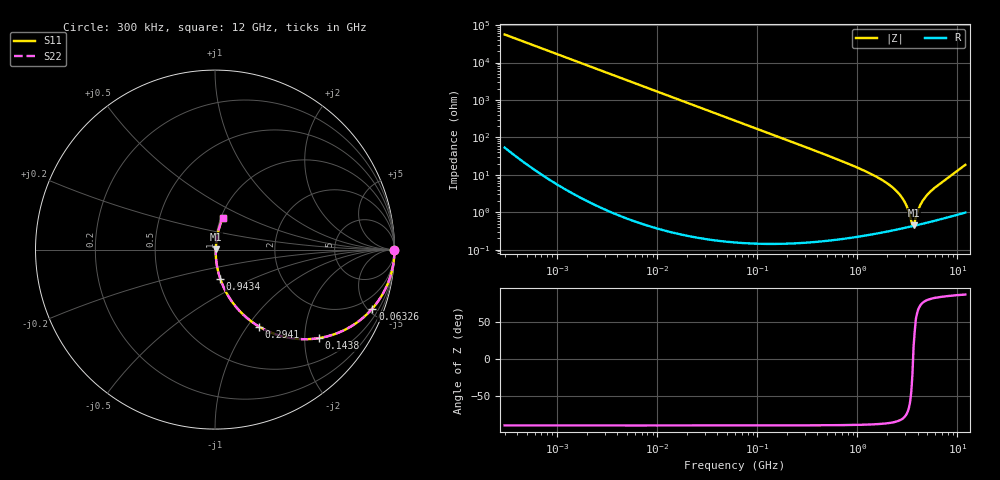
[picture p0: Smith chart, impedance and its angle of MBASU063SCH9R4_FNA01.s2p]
! MBASU063SCH9R4_FNA01  S-PARAMETER MODEL  ( General Type )
! Model Generated by TAIYO YUDEN Corporation (http://www.ty-top.com)
! Version 1.0
! TAIYO YUDEN Control No. 130801
! Copyright(c) 2013 TAIYO YUDEN CO.,LTD. All Rights Reserved.
! Product Description (link to TY-COMPAS)
! https://ds.yuden.co.jp/TYCOMPAS/or/detail?pn=MBASU063SCH9R4DFNA01&u=M
! Products Name : Multilayer Ceramic Capacitors
! Characteristics :
!  Capacitance : 9.4 pF , Rated Voltage : 50V , TCC : CH / C0H
!  Case Size : 0.6 x 0.3 / 0.024 x 0.012 [mm/inch] , Thickness : 0.3 / 0.012 [mm/inch]
!  (Conditions: Temperature = 25 degC , DC Bias Current/Voltage = 0A / 0V)
! External Node Assignments :
!  1  o---| |---o  2
! GND o---------o GND
! Frequency Range : 0.3MHz  -  12000MHz  [ 401 STEP ]
# MHz S RI R 50
! Freq[MHz].  S11 Real  S11 Imag  S21 Real  S21 Imag  S12 Real  S12 Imag  S22 Real  S22 Imag
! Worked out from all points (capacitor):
!   401 points, 300 kHz to 12 GHz, reference 50 ohm
!   read as one part in series: C = 9.42 pF near 316.3 kHz
!   lowest |Z| = 449 mohm at 3.643 GHz (marker M1)
!   series resonance near 3.603 GHz, so ESL is about 210 pH
!   S11 on the Smith chart (normalised r, x): 300 kHz: open; 63.26 MHz: 1.00, -5.34; 143.8 MHz: 1.00, -2.35; 294.1 MHz: 1.00, -1.14; 943.4 MHz: 1.00, -0.33; 12 GHz: 1.02, +0.37
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0.3  1 -0.00177  4.84e-06 0.00177  4.84e-06 0.00177  1 -0.00177
1.769972  0.9999 -0.0105  0.000112 0.0105  0.000112 0.0105  0.9999 -0.0105
10.44266  0.9962 -0.0615  0.00382 0.0615  0.00382 0.0615  0.9962 -0.0615
26.39317  0.9762 -0.1524  0.0238 0.1524  0.0238 0.1524  0.9762 -0.1524
60  0.8879 -0.3152  0.1121 0.3152  0.1121 0.3152  0.8879 -0.3152
63.26471  0.8769 -0.3282  0.1231 0.3282  0.1231 0.3282  0.8769 -0.3282
94.13233  0.7629 -0.4249  0.2371 0.4249  0.2371 0.4249  0.7629 -0.4249
143.8206  0.5792 -0.4931  0.4208 0.4931  0.4208 0.4931  0.5792 -0.4931
294.0765  0.2465 -0.4296  0.7535 0.4296  0.7535 0.4296  0.2465 -0.4296
353.9943  0.1836 -0.3855  0.8164 0.3855  0.8164 0.3855  0.1836 -0.3855
555.3718  0.0825 -0.2722  0.9175 0.2722  0.9175 0.2722  0.0825 -0.2722
943.3804  0.0291 -0.1618  0.9709 0.1618  0.9709 0.1618  0.0291 -0.1618
1519.776  0.0109 -0.0903  0.9891 0.0903  0.9891 0.0903  0.0109 -0.0903
2088.533  0.00599 -0.0534  0.994 0.0534  0.994 0.0534  0.00599 -0.0534
2795.104  0.00425 -0.024  0.9957 0.024  0.9957 0.024  0.00425 -0.024
3107.553  0.0041 -0.014  0.9959 0.014  0.9959 0.014  0.0041 -0.014
3454.93  0.00418 -0.0041  0.9958 0.0041  0.9958 0.0041  0.00418 -0.0041
3642.919  0.0043 0.00123  0.9957 -0.00123  0.9957 -0.00123  0.0043 0.00123
3740.715  0.00438 0.00329  0.9956 -0.00329  0.9956 -0.00329  0.00438 0.00329
4270.516  0.00498 0.0151  0.995 -0.0151  0.995 -0.0151  0.00498 0.0151
5140.631  0.00631 0.0308  0.9937 -0.0308  0.9937 -0.0308  0.00631 0.0308
12000  0.042 0.1758  0.958 -0.1758  0.958 -0.1758  0.042 0.1758
